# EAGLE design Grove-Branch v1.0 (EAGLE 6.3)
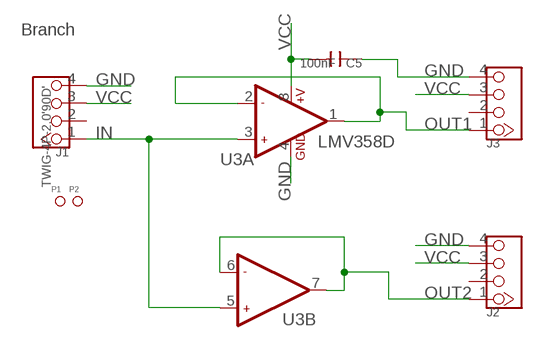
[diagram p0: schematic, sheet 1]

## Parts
C5  100nF  C-0603  [C0603]
J1  TWIG-4P-2.0'90D'  [4P-2.0-90D]
J2  TWIG-4P-2.0'90D'  [4P-2.0-90D]
J3  TWIG-4P-2.0'90D'  [4P-2.0-90D]
P1  PAD-MARK  [ROUND-MARK-1.0]
P2  PAD-MARK  [ROUND-MARK-1.0]
U3  LMV358D  [SO08]

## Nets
GND: C5.1 J1.4 J2.4 J3.4 U3.4(A:GND)
IN: J1.1 U3.3(A:+IN1) U3.5(B:+IN2)
OUT1: J3.1 U3.1(A:OUT1) U3.2(A:-IN1)
OUT2: J2.1 U3.6(B:-IN2) U3.7(B:OUT2)
VCC: C5.2 J1.3 J2.3 J3.3 U3.8(A:+V)
Unconnected: J1.2 J2.2 J3.2

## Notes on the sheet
- Branch

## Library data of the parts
C5 = Discrete:C*: Ceramic Capacitors
J1-J3 = Connector:TWIG-4P-2.0
P1 P2 = Discrete:PAD-MARK; PARTNO: DNP
U3 = IC:LMV358: General purpose LOW Voltage, Rail-to-Rail Output Amplifiers http://www.fairchildsemi.com/ds/LM/LMV358.pdf

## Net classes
0 default: width 0.152 mm, drill 0.305 mm, clearance 0.152 mm

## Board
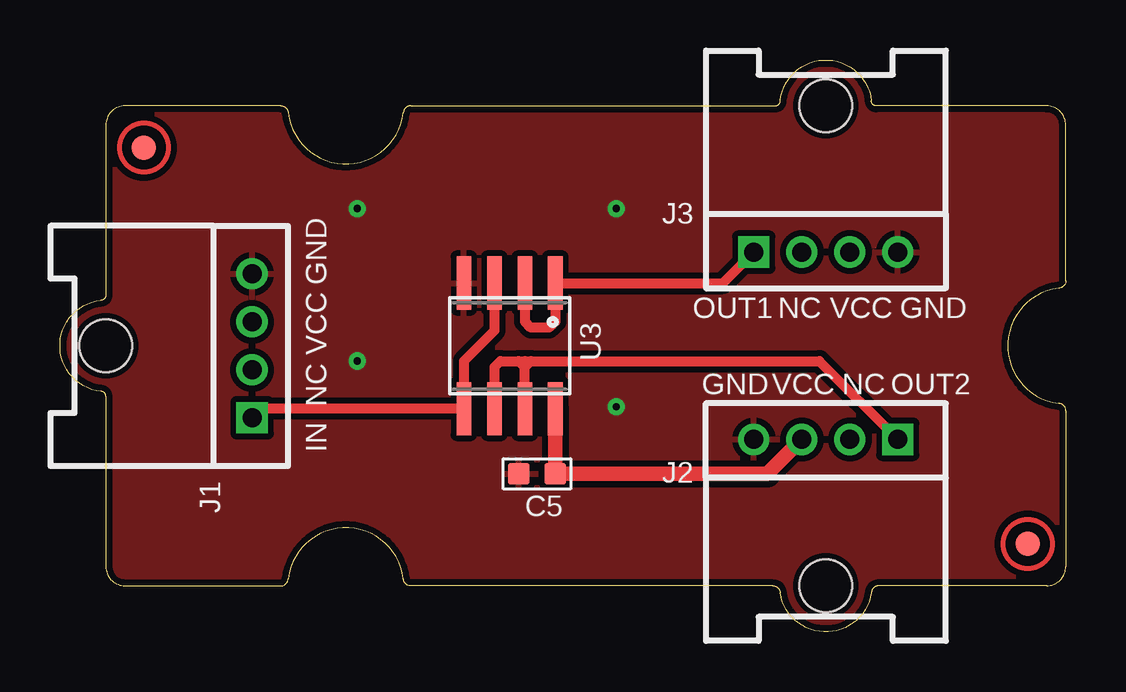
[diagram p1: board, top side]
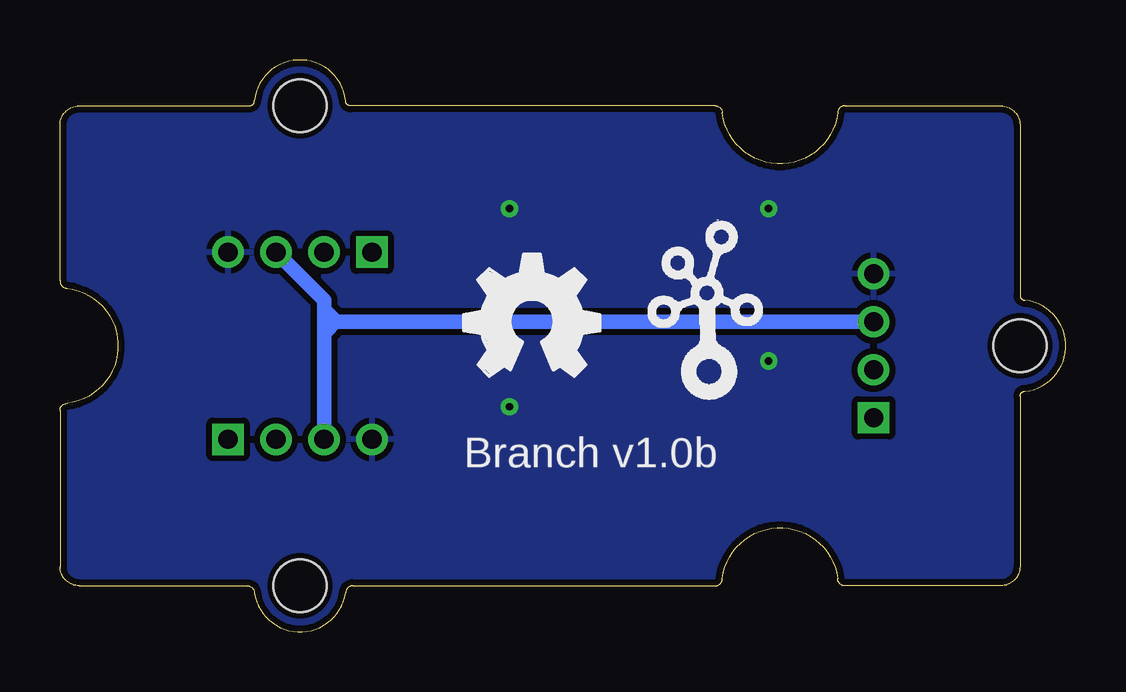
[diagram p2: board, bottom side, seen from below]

Size 41.91 x 23.83 mm. Coordinates in mm from the lower left corner, seen from the top.
Copper layers (1*16): Top 0.035mm / dielectric 1.5mm / Bottom 0.035mm
Design rules "default": minimum track width 10mil, minimum drill 10mil, track to track 8mil, track to pad 8mil, pad to pad 8mil, via to via 8mil, smd to smd 0mil, copper to edge 10mil, drill to drill 8mil, minimum pad ring 10mil, minimum via ring 8mil, stop-mask expansion 4mil, vias tented up to drill 25mil, thermal gap 10mil

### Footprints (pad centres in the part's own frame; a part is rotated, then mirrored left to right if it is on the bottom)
C0603 = smd 0.889 x 0.889: 1 -0.762,0; 2 0.762,0
4P-2.0-90D = drill 0.8 pad 1.27 square: 1 -3,0 | drill 0.8 pad 1.27: 2 -1,0; 3 1,0; 4 3,0
ROUND-MARK-1.0 = smd 1.016 x 1.016: P$1 0,0
SO08 = smd 0.61 x 2.21: 1 -1.905,-2.616; 2 -0.635,-2.616; 3 0.635,-2.616; 4 1.905,-2.616; 5 1.905,2.616; 6 0.635,2.616; 7 -0.635,2.616; 8 -1.905,2.616
2U-DIM-W/DRILL = hole 2.2: -10,-10; -10,10; 20,0

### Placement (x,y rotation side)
C5  19.88,6.59 0 top
J1  8.01,11.92 90 top
J2  31.91,8.02 180 top
J3  31.91,15.82 0 top
P1  3.49,20.18 0 top
P2  40.32,3.67 0 top
U3  18.73,11.92 180 top
U$1  [2U-DIM-W/DRILL]  21.91,11.92 180 top
U$2  [OSHW_FILLX200_NOTEXT]  25.08,10.65 0 bottom
U$3  [TWIGLOGO]  14.92,10.65 0 bottom

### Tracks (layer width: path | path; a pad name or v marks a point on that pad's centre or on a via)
GND  (via drill 0.3 pad 0.64)
  other vias: 23.18,17.64 23.18,9.38 12.38,17.64 12.38,11.29
  pour Top (isolate 0.254): -0.32,23.99 42.86,23.99 42.86,-0.14 -0.32,-0.14
  pour Bottom (isolate 0.254): -0.32,23.99 -0.32,-0.14 42.86,-0.14 42.86,23.99
IN
  Top 0.406: J1.1 8.39,9.31 U3.5 16.83,11.29 18.1,12.56 U3.3
OUT1
  Top 0.406: J3.1 27.62,14.54 U3.1 20.64,12.94 20.38,12.68 19.62,12.68 19.37,12.94 U3.2
OUT2
  Top 0.406: 19.37,11.29 19.62,11.29 | 19.62,11.29 31.64,11.29 J2.1 | U3.7 19.37,11.03 | 19.37,11.03 19.37,11.29 | 19.11,11.29 18.35,11.29 18.1,11.03 U3.6 | 19.11,11.29 19.37,11.29 | 19.37,11.03 19.11,11.29 | 19.37,11.03 19.62,11.29
VCC
  Top 0.61: U3.8 C5.2 29.47,6.59 J2.3
  Bottom 0.61: J2.3 30.91,12.81 | 30.91,12.81 30.91,13.82 J3.3 | J1.3 30.4,12.92 | 30.43,12.92 30.8,12.92 30.91,12.81 | 30.4,12.92 30.8,13.32 | 30.4,12.92 30.43,12.92 | 30.43,12.92 30.8,12.56

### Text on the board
tPlace: GND | OUT1 | NC | VCC | GND | VCC | GND | VCC | NC | OUT2 | NC | IN
bPlace: Branch v1.0b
